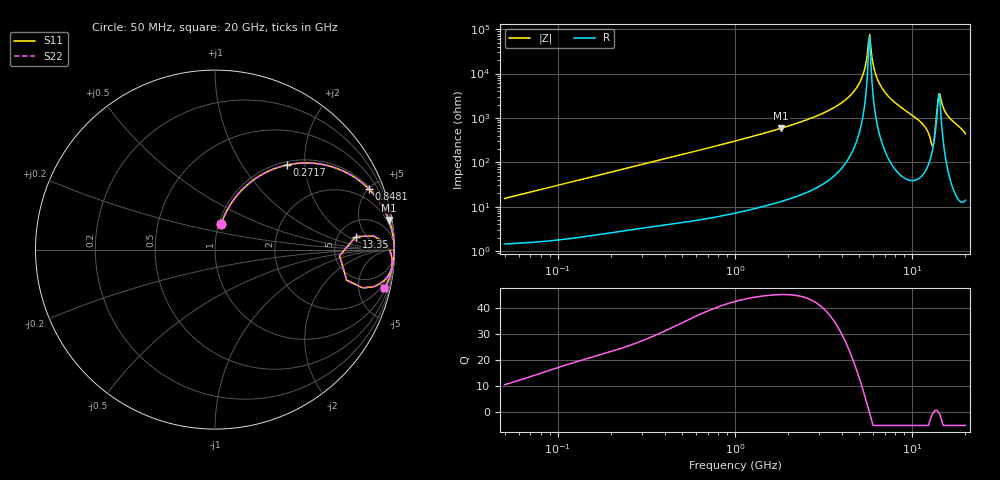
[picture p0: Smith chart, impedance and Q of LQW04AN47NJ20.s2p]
!Murata Part Number: LQW04AN47NJ20
!These Parameters are Measured in Series Mode Connection
!  o--[Z]--o
!Port1  Port2
!  o-------o
!Freq. Start=50[MHz] Stop=20[GHz], 401[Steps]
# Hz S RI R 50
!Freq.(Hz) S11(Real) S11(Imag) S21(Real) S21(Imag) S12(Real) S12(Imag) S22(Real) S22(Imag)
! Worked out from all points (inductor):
!   401 points, 50 MHz to 20 GHz, reference 50 ohm
!   read as one part in series: L = 48.2 nH near 51.52 MHz
!   highest Q = 44.9 at 1.821 GHz (marker M1), where L = 51.1 nH
!   self-resonance near 5.683 GHz
!   S11 on the Smith chart (normalised r, x): 50 MHz: 1.03, +0.30; 271.7 MHz: 1.06, +1.62; 848.1 MHz: 1.12, +5.06; 13.35 GHz: 7.37, +2.84; 20 GHz: 1.28, -8.76
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5e7  0.0357 0.1441  0.9643 -0.1441  0.9643 -0.1441  0.0357 0.1441
1.364002e8  0.1565 0.3391  0.8435 -0.3391  0.8435 -0.3391  0.1565 0.3391
2.716764e8  0.3993 0.4711  0.6007 -0.4711  0.6007 -0.4711  0.3993 0.4711
3.721004e8  0.5476 0.4814  0.4524 -0.4814  0.4524 -0.4814  0.5476 0.4814
8.480927e8  0.8591 0.3359  0.1409 -0.3359  0.1409 -0.3359  0.8591 0.3359
1e9  0.8948 0.2953  0.1052 -0.2953  0.1052 -0.2953  0.8948 0.2953
1.820564e9  0.9681 0.1649  0.0319 -0.1649  0.0319 -0.1649  0.9681 0.1649
2.728004e9  0.988 0.0977  0.012 -0.0977  0.012 -0.0977  0.988 0.0977
4.677679e9  0.998 0.0256  0.00199 -0.0256  0.00199 -0.0256  0.998 0.0256
5.194772e9  0.9986 0.0126  0.0014 -0.0126  0.0014 -0.0126  0.9986 0.0126
5.433528e9  0.9987 0.00697  0.00127 -0.00697  0.00127 -0.00697  0.9987 0.00697
5.598765e9  0.9988 0.00323  0.00122 -0.00323  0.00122 -0.00323  0.9988 0.00323
5.769027e9  0.9988 -0.000534  0.0012 0.000534  0.0012 0.000534  0.9988 -0.000534
6.406762e9  0.9986 -0.0139  0.00138 0.0139  0.00138 0.0139  0.9986 -0.0139
7.442007e9  0.9975 -0.0342  0.00247 0.0342  0.00247 0.0342  0.9975 -0.0342
1.149051e10  0.9721 -0.1327  0.0279 0.1327  0.0279 0.1327  0.9721 -0.1327
1.276073e10  0.8226 -0.2131  0.1774 0.2131  0.1774 0.2131  0.8226 -0.2131
1.334722e10  0.7857 0.0726  0.2143 -0.0726  0.2143 -0.0726  0.7857 0.0726
1.396067e10  0.9597 0.0192  0.0403 -0.0192  0.0403 -0.0192  0.9597 0.0192
1.438523e10  0.9798 -0.0213  0.0202 0.0213  0.0202 0.0213  0.9798 -0.0213
1.597544e10  0.9866 -0.0898  0.0134 0.0898  0.0134 0.0898  0.9866 -0.0898
2e10  0.9444 -0.2139  0.0556 0.2139  0.0556 0.2139  0.9444 -0.2139
